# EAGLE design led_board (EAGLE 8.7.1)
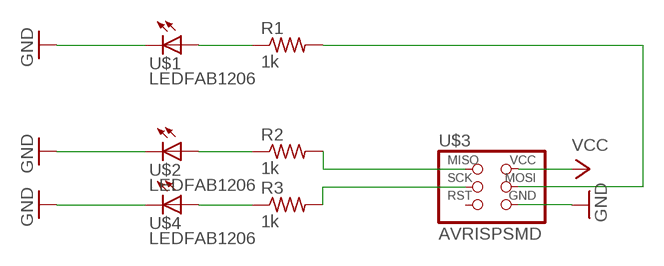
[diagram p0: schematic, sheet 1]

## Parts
R1  1k  RES-US1206FAB  [R1206FAB]
R2  1k  RES-US1206FAB  [R1206FAB]
R3  1k  RES-US1206FAB  [R1206FAB]
U$1  LEDFAB1206  [LED1206FAB]
U$2  LEDFAB1206  [LED1206FAB]
U$3  AVRISPSMD  [2X03SMD]
U$4  LEDFAB1206  [LED1206FAB]

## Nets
GND: U$1.2(C) U$2.2(C) U$3.6(GND) U$4.2(C)
N$1: R1.1 U$1.1(A)
N$2: R1.2 U$3.4(MOSI)
N$3: R2.1 U$2.1(A)
N$4: R3.1 U$4.1(A)
N$5: R2.2 U$3.1(MISO)
N$6: R3.2 U$3.3(SCK)
VCC: U$3.2(VCC)
Unconnected: U$3.5(RST)

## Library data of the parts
R1-R3 = fab:RES-US: Resistor (US Symbol)
U$1 U$2 U$4 = fab:LED: LED
U$3 = fab:AVRISP

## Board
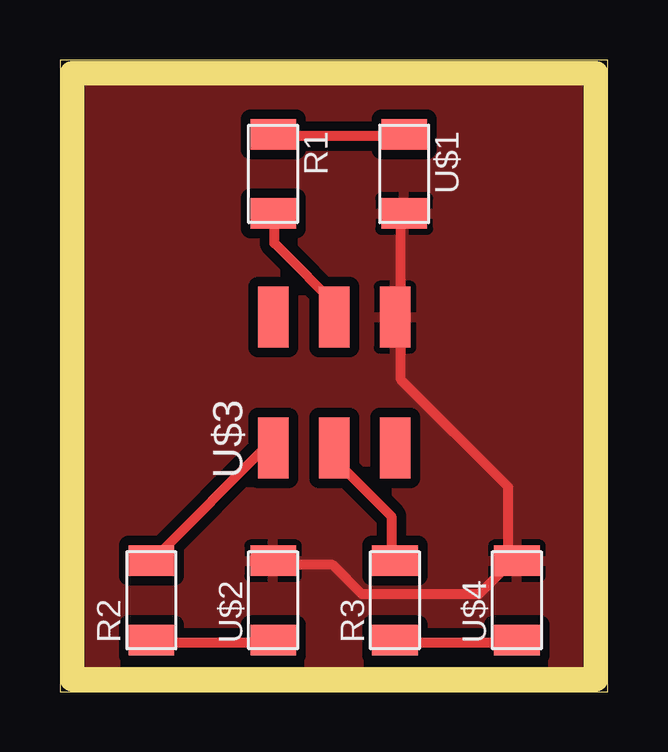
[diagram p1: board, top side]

Size 22.84 x 26.34 mm. Coordinates in mm from the lower left corner, seen from the top.
Outline: 0,0 22.84,0 22.84,26.34 0,26.34 0,0
Copper layers (1*16): Top 0.035mm / dielectric 1.5mm / Bottom 0.035mm
Design rules "default *": minimum track width 16mil, minimum drill 0.35mm, track to track 16mil, track to pad 16mil, pad to pad 16mil, via to via 16mil, smd to smd 16mil, copper to edge 40mil, drill to drill 6mil, minimum pad ring 10mil, minimum via ring 8mil, stop-mask expansion 4mil, vias tented up to drill 0mil, thermal gap 10mil
Milling: 4 lines

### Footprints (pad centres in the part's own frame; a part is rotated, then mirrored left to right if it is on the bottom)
R1206FAB = smd 1.27 x 1.905: 1 -1.651,0; 2 1.651,0
LED1206FAB = smd 1.27 x 1.905: 1 -1.651,0; 2 1.651,0
2X03SMD = smd 2.54 x 1.27: 1 -2.54,2.54; 2 2.92,2.54; 3 -2.54,0; 4 2.92,0; 5 -2.54,-2.54; 6 2.92,-2.54

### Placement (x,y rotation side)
R1  8.89,21.59 270 top
R2  3.81,3.81 90 top
R3  13.97,3.81 90 top
U$1  14.35,21.59 270 top
U$2  8.89,3.81 90 top
U$3  11.43,12.7 90 top
U$4  19.05,3.81 90 top

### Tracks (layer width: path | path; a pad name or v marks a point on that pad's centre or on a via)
GND
  Top 0.406: U$1.2 14.22,19.91 14.22,15.85 U$3.6 14.22,15.44 14.22,13.01 18.69,8.53 18.69,5.69 U$4.2 18.69,5.28 17.48,4.06 12.6,4.06 11.38,5.28 8.94,5.28 U$2.2
  pour Top: 0,25.4 22.86,25.4 22.86,0 0,0
N$1
  Top 0.406: R1.1 8.94,23.16 14.22,23.16 U$1.1
N$2
  Top 0.406: R1.2 8.94,19.91 8.94,18.69 11.79,15.85 U$3.4
N$3
  Top 0.406: R2.1 4.06,2.03 8.53,2.03 U$2.1
N$4
  Top 0.406: R3.1 14.22,2.03 18.69,2.03 U$4.1
N$5
  Top 0.406: R2.2 4.06,5.69 8.53,10.16 U$3.1
N$6
  Top 0.406: R3.2 13.82,5.69 13.82,7.32 11.79,9.35 11.79,10.16 U$3.3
